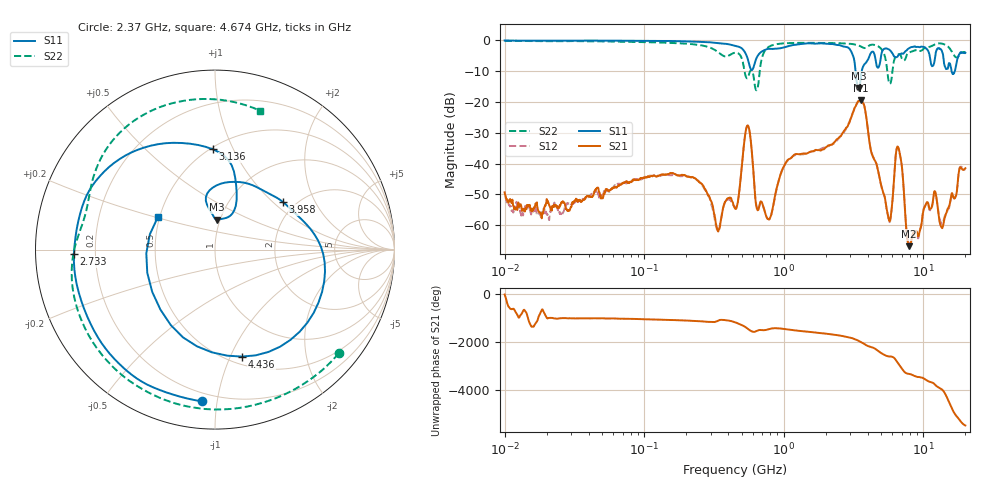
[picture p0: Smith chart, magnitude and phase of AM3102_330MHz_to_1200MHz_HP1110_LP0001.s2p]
! Date/Time: Tue, Sep 11, 2018 5:23 PM
! Network Analyzer: Agilent Technologies E8362B Rev: A.07.50.63
! Sweep from 0.010 to 20.000 GHz, 1601 Points, Sweep Type: LOG
! Power Supply: 4.949 V, 0.001 A
# Hz S DB R 50
!freq MagS11 AngS11 MagS21 AngS21 MagS12 AngS12 MagS22 AngS22
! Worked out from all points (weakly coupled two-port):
!   1601 points, 10 MHz to 20 GHz, reference 50 ohm
!   highest |S21| = -19.44 dB at 3.549 GHz (marker M1); lowest = -66.8 dB at 7.882 GHz (marker M2)
!   lowest |S11| = -15.5 dB at 3.449 GHz (marker M3), VSWR 1.40, Z = 48.3 + j16.6 ohm
!   |S11| at or under -10 dB: 3.266 GHz to 3.618 GHz (351.4 MHz wide, 10.2 % of centre); 15.92 GHz to 16.8 GHz (887.7 MHz wide, 5.43 % of centre)
!   |S22| runs from -16.2 to -0.2 dB; largest |S21 - S12| = 0.0059
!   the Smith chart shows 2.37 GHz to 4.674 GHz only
!   S11 on the Smith chart (normalised r, x): 2.37 GHz: 0.15, -0.91; 2.733 GHz: 0.12, -0.02; 3.136 GHz: 0.51, +0.84; 3.958 GHz: 1.71, +1.16; 4.436 GHz: 0.58, -1.11; 4.674 GHz: 0.49, +0.21
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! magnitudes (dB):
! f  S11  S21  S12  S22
! 10 MHz  0.0  -49.4  -50.8  -0.2
! 35.55 MHz  -0.1  -52.3  -51.7  -0.3
! 126.4 MHz  -0.2  -44.0  -44.0  -0.7
! 248.1 MHz  -0.5  -46.1  -45.9  -1.5
! 334.7 MHz  -0.9  -61.5  -61.9  -3.7
! 447.2 MHz  -1.8  -54.5  -54.2  -4.0
! 548.6 MHz  -5.7  -27.7  -27.7  -12.3
! 641.7 MHz  -5.5  -54.7  -54.3  -16.1
! 772.3 MHz  -2.8  -58.0  -58.0  -2.3
! 1.59 GHz  -1.0  -36.1  -36.0  -0.8
! 2.37 GHz  -1.4  -32.4  -32.8  -0.9
! 2.733 GHz  -2.1  -29.1  -29.5  -1.0
! 3.136 GHz  -5.0  -23.4  -23.4  -1.2
! 3.449 GHz  -15.5  -19.7  -19.7  -1.7
! 3.549 GHz  -12.7  -19.4  -19.4  -2.0
! 3.958 GHz  -6.7  -27.3  -27.2  -2.1
! 4.436 GHz  -4.2  -38.6  -38.5  -1.5
! 4.674 GHz  -8.7  -41.2  -41.2  -1.8
! 5.652 GHz  -2.9  -58.2  -58.4  -13.5
! 6.612 GHz  -4.8  -34.8  -34.9  -4.6
! 7.882 GHz  -2.6  -66.8  -66.4  -4.0
! 20 GHz  -4.1  -41.5  -42.0  -3.8
